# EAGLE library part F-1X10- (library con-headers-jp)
FEMALE HEADER
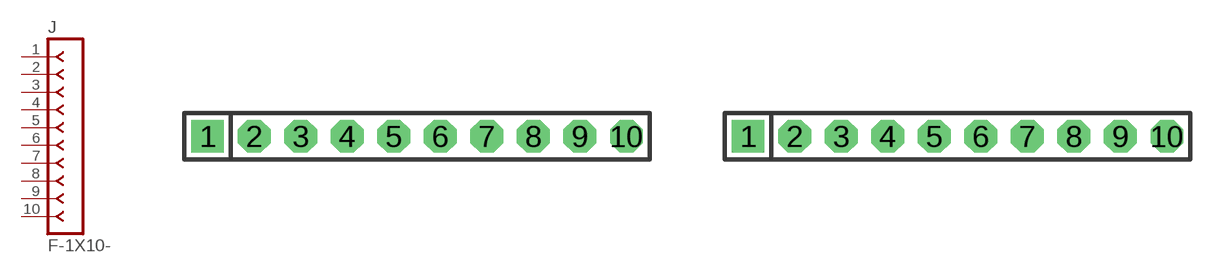
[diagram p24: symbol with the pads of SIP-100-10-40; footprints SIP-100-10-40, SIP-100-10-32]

Designator prefix J

## F-1X10-SIP-100-40  [SIP-100-10-40]
1  1  pas
2  2  pas
3  3  pas
4  4  pas
5  5  pas
6  6  pas
7  7  pas
8  8  pas
9  9  pas
10  10  pas

## F-1X10-SIP-100-32  [SIP-100-10-32]
Pads as for SIP-100-10-40

## F-1X10-SIP-100-32Y  [SIP-100-10-32Y]
Pads as for SIP-100-10-40

## F-1X10-SIP-100-40Y  [SIP-100-10-40Y]
Pads as for SIP-100-10-40

## F-1X10-KK-4455-B10  [KK-4455-B10]
Pads as for SIP-100-10-40

## F-1X10-KK-4455-C10  [KK-4455-C10]
Pads as for SIP-100-10-40

## F-1X10-KK-4455-A10  [KK-4455-A10]
Pads as for SIP-100-10-40

## Footprint SIP-100-10-40 (pad centres in mm)
SIP Header - 0.1", 40 mil drill
drill 1.016 pad 1.778 square: 1 -11.43,0
drill 1.016 pad 1.778 octagon: 2 -8.89,0; 3 -6.35,0; 4 -3.81,0; 5 -1.27,0; 6 1.27,0; 7 3.81,0; 8 6.35,0; 9 8.89,0; 10 11.43,0

## Footprint SIP-100-10-32 (pad centres in mm)
SIP Header - 0.1", 32 mil drill
drill 0.813 pad 1.778 square: 1 -11.43,0
drill 0.813 pad 1.778 octagon: 2 -8.89,0; 3 -6.35,0; 4 -3.81,0; 5 -1.27,0; 6 1.27,0; 7 3.81,0; 8 6.35,0; 9 8.89,0; 10 11.43,0

## Footprint SIP-100-10-32Y (pad centres in mm)
SIP Header - 0.1", 32 mil drill
drill 0.813 long: 1 -11.43,0; 2 -8.89,0; 3 -6.35,0; 4 -3.81,0; 5 -1.27,0; 6 1.27,0; 7 3.81,0; 8 6.35,0; 9 8.89,0; 10 11.43,0

## Footprint SIP-100-10-40Y (pad centres in mm)
SIP Header - 0.1", 40 mil drill
drill 1.016 long: 1 -11.43,0; 2 -8.89,0; 3 -6.35,0; 4 -3.81,0; 5 -1.27,0; 6 1.27,0; 7 3.81,0; 8 6.35,0; 9 8.89,0; 10 11.43,0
